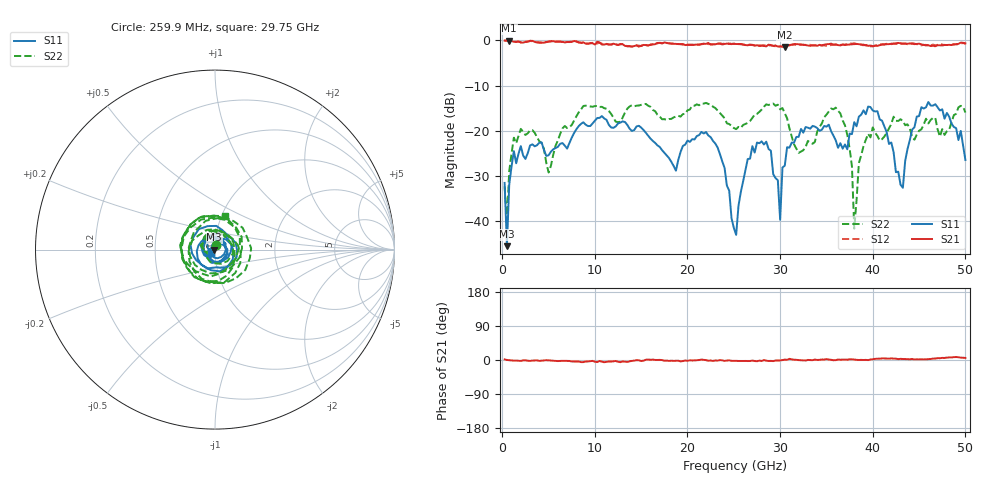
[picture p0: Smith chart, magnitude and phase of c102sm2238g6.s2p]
! 12/2/2019 9:38:22 AM
! Y:\TERRY-ANALYZER-FILES\DON MINNICK\C102SM2238G6.S2P
! CHANNEL.1
! TR.MEASUREMENT
! CORRECTED.DATA
# GHZ S RI R 50.0
! FREQ.GHZ  S11RE  S11IM  S21RE  S21IM  S12RE  S12IM  S22RE  S22IM
!; PortSelection: Port_12
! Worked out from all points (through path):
!   200 points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, 259.9 MHz to 50 GHz, reference 50 ohm
!   highest |S21| = -0.03 dB at 759.9 MHz (marker M1); lowest = -1.5 dB at 30.5 GHz (marker M2)
!   lowest |S11| = -45.5 dB at 509.9 MHz (marker M3), VSWR 1.01, Z = 49.5 - j0.0451 ohm
!   |S11| at or under -10 dB: start of sweep to end of sweep
!   |S22| runs from -41.6 to -13.8 dB; largest |S21 - S12| = 0.045
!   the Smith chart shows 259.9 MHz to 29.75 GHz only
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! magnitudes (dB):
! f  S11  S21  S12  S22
! 259.9 MHz  -31.5  0.0  0.0  -32.3
! 509.9 MHz  -45.5  0.0  0.0  -39.8
! 759.9 MHz  -31.9  0.0  0.0  -28.9
! 2.01 GHz  -23.4  -0.5  -0.4  -19.6
! 5.009 GHz  -25.4  -0.2  -0.3  -29.2
! 8.758 GHz  -18.1  -0.4  -0.6  -14.5
! 17.01 GHz  -23.6  -0.5  -0.5  -16.9
! 22.51 GHz  -21.4  -0.9  -0.8  -14.2
! 25.25 GHz  -43.0  -0.8  -0.8  -19.6
! 27 GHz  -23.4  -1.0  -1.0  -17.1
! 29 GHz  -24.4  -1.0  -1.1  -14.2
! 30 GHz  -39.7  -1.3  -1.3  -15.3
! 30.5 GHz  -27.7  -1.5  -1.4  -16.1
! 33.5 GHz  -18.9  -1.0  -1.1  -22.9
! 36.5 GHz  -22.8  -1.1  -1.0  -16.2
! 37.75 GHz  -20.7  -0.9  -0.7  -27.8
! 38 GHz  -18.1  -0.8  -0.6  -41.6
! 39 GHz  -15.5  -0.9  -1.1  -23.4
! 41.75 GHz  -22.9  -0.8  -0.7  -19.5
! 43.25 GHz  -32.6  -0.7  -0.8  -17.8
! 46 GHz  -13.6  -1.1  -1.1  -18.4
! 50 GHz  -26.5  -0.7  -0.7  -16.0
